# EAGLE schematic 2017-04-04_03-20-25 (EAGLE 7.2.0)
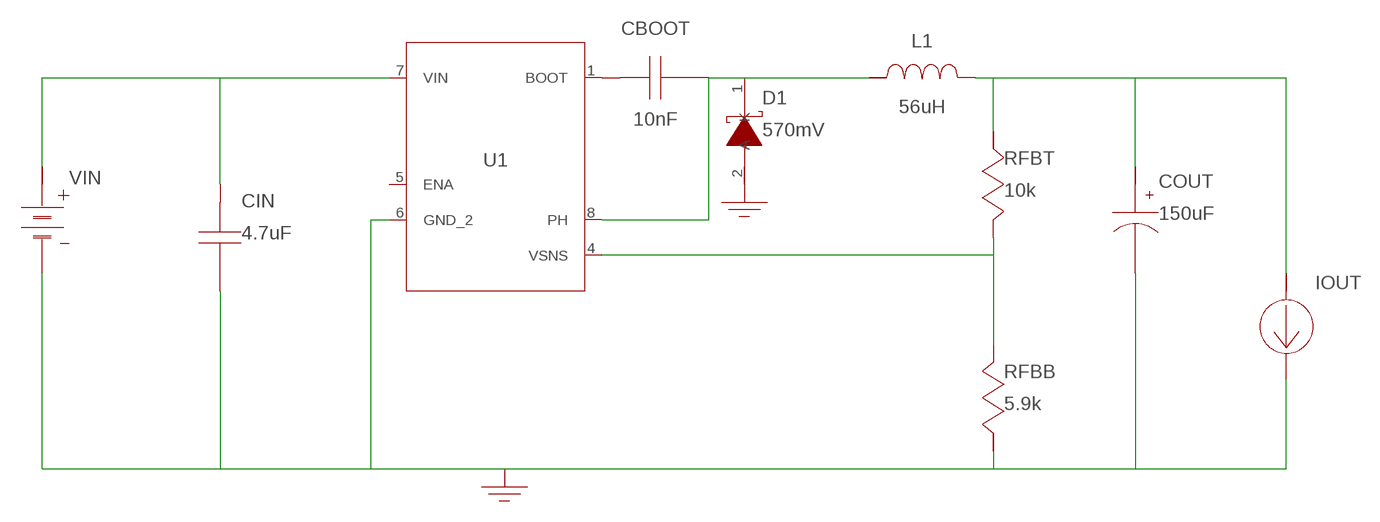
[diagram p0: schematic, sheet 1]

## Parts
CBOOT  10nF  CGA2B3X7R1H103K050BB  [0402]
CIN  4.7uF  GRM31CR71H475KA12L  [1206]
COUT  150uF  4TPH150MABC  [CAPSMT_6_A14]
D1  570mV  PMEG6010CEH,115  [SOD-123F]
GND  WB_GND  WB_GNDWB_GND  [WB_GND]
GND5  WB_GND  WB_GNDWB_GND  [WB_GND]
IOUT  WB_CURRENT_LOAD  WB_CURRENT_LOADWB_CURRENT_LOAD  [WB_CURRENT_LOAD]
L1  56uH  NPI75C560KTRF  [IND_NPI75C]
RFBB  5.9k  CRCW04025K90FKED  [0402]
RFBT  10k  CRCW040210K0FKED  [0402]
U1  TPS5410DR  [M08A]
VIN  WB_BATTERY  WB_BATTERYWB_BATTERY  [WB_BATTERY]

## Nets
0: CIN.2 COUT.2(-) D1.2(A) GND5.1 GND.1 IOUT.2(-) RFBB.2 U1.6(GND_2) VIN.2(-)
2: CBOOT.2 D1.1(K) L1.2 U1.8(PH)
3: RFBB.1 RFBT.1 U1.4(VSNS)
4: CIN.1 U1.7(VIN) VIN.1(+)
5: COUT.1(+) IOUT.1(+) L1.1 RFBT.2
6: CBOOT.1 U1.1(BOOT)
Unconnected: U1.5(ENA)

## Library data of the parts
CBOOT = AcceleratedDesigns_Lib:CGA2B3X7R1H103K050BB; CAP: 1.0E8; DATASHEETURL: httpsproduct.tdk.comensearchcapacitorceramicmlccinfo?part%5Fno%3DCGA2B3X7R1H103K050BB; ESR: 0.333065; IRMS: 0.323373; MANUFACTURER_NAME: TDK; MANUFACTURER_PART_NUMBER: CGA2B3X7R1H103K050BB; VDC: 50.0; VENDOR: TDK
CIN = AcceleratedDesigns_Lib:GRM31CR71H475KA12L; CAP: 4.7E6; ESR: 0.0; IRMS: 0.0; MANUFACTURER_NAME: MuRata; MANUFACTURER_PART_NUMBER: GRM31CR71H475KA12L; VDC: 50.0; VENDOR: MuRata
COUT = AcceleratedDesigns_Lib:4TPH150MABC; CAP: 1.5E4; DATASHEETURL: httpindustrial.panasonic.comwww%2DdatapdfAAA8000AAA8000CE2.pdf; ESR: 0.07; IRMS: 0.74; MANUFACTURER_NAME: Panasonic; MANUFACTURER_PART_NUMBER: 4TPH150MABC; VDC: 4.0; VENDOR: Panasonic
D1 = AcceleratedDesigns_Lib:PMEG6010CEH,115; DATASHEETURL: httpwww.nxp.comdocumentsdata%5FsheetPMEG6010CEH%5FPMEG6010CEJ.pdf; IO: 1.0; MANUFACTURER_NAME: Nexperia; MANUFACTURER_PART_NUMBER: PMEG6010CEH115; VENDOR: NXP Semiconductor; VFATIO: 0.57; VRRM: 60.0
GND GND5 = AcceleratedDesigns_Lib:WB_GND; MANUFACTURER_NAME: WB_GND; MANUFACTURER_PART_NUMBER: WB_GND; POWERPORTTYPE: POWER_GROUND; VALUE: Value
IOUT = AcceleratedDesigns_Lib:WB_CURRENT_LOAD; MANUFACTURER_NAME: WB_CURRENT_LOAD; MANUFACTURER_PART_NUMBER: WB_CURRENT_LOAD; POWERPORTTYPE: POWER_GROUND; VALUE: Value
L1 = AcceleratedDesigns_Lib:NPI75C560KTRF; DCR: 0.24; IDC: 0.94; L: 5.6E5; MANUFACTURER_NAME: NIC Components; MANUFACTURER_PART_NUMBER: NPI75C560KTRF; VENDOR: NIC Components
RFBB = AcceleratedDesigns_Lib:CRCW04025K90FKED; MANUFACTURER_NAME: VishayDale; MANUFACTURER_PART_NUMBER: CRCW04025K90FKED; POWER: 0.063; RESISTANCE: 5900.0; TOLERANCE: 1.0; VENDOR: VishayDale
RFBT = AcceleratedDesigns_Lib:CRCW040210K0FKED; MANUFACTURER_NAME: VishayDale; MANUFACTURER_PART_NUMBER: CRCW040210K0FKED; POWER: 0.063; RESISTANCE: 10000.0; TOLERANCE: 1.0; VENDOR: VishayDale
U1 = AcceleratedDesigns_Lib:TPS5410DR; DATASHEETURL: httpwww.ti.comproducttps5410; FREQUENCY: 500000.0; IMAX: 1.0; MANUFACTURER_NAME: Texas Instruments; MANUFACTURER_PART_NUMBER: TPS5410DR; MKTG_PACKAGE: TPS5410; NSID: TPS5410D; PACKAGE: TPS5410; VENDOR: Texas Instruments
VIN = AcceleratedDesigns_Lib:WB_BATTERY; MANUFACTURER_NAME: WB_BATTERY; MANUFACTURER_PART_NUMBER: WB_BATTERY; POWERPORTTYPE: POWER_GROUND; VALUE: Value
